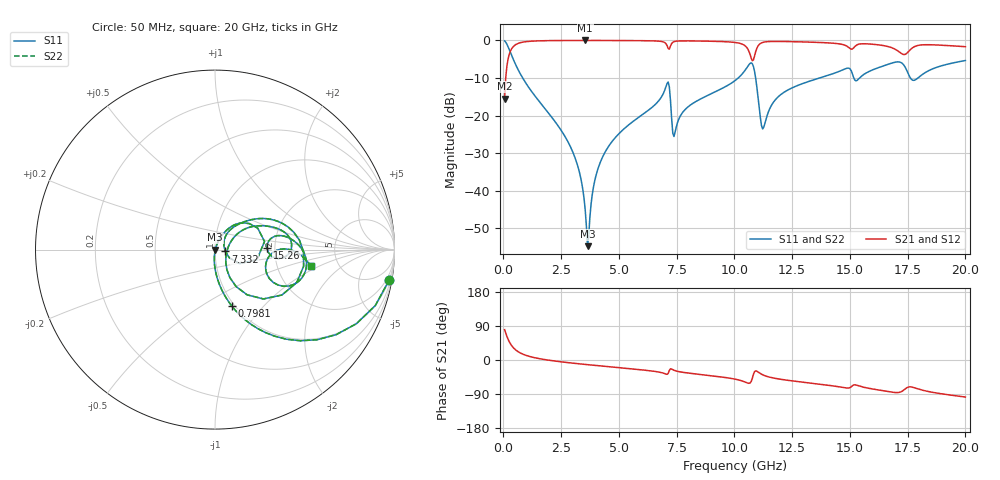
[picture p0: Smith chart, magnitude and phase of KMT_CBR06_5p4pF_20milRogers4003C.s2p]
! Data measured by Modelithics Inc. support@modelithics.com 813-866-6335
! KEMET CBR0603 5.4pF, Pad Width= 0.851mm, Pad Length= 0.64mm, Pad Gap= 0.62mm, 20mil Rogers 4003C substrate Data, January 2022
# hz S ma R 50
! 2 Port Network Data from SP1.SP block
! freq  magS11  angS11  magS21  angS21  magS12  angS12  magS22  angS22
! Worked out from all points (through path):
!   401 points, 50 MHz to 20 GHz, reference 50 ohm
!   highest |S21| = -0.02 dB at 3.541 GHz (marker M1); lowest = -15.5 dB at 50 MHz (marker M2)
!   group delay of S21, straight-line fit = 15.3 ps
!   lowest |S11| = -54.7 dB at 3.641 GHz (marker M3), VSWR 1.00, Z = 50.2 - j0.0924 ohm
!   |S11| at or under -10 dB: 833 MHz to 10.16 GHz (9.33 GHz wide, 170 % of centre); 10.92 GHz to 13.68 GHz (2.766 GHz wide, 22.5 % of centre); 17.62 GHz to 17.95 GHz (322.8 MHz wide, 1.82 % of centre)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
!   |S22| runs from -54.7 to -0.1 dB; largest |S21 - S12| = 0
!   S11 on the Smith chart (normalised r, x): 50 MHz: 1, -11; 798.1 MHz: 0.97, -0.69; 7.332 GHz: 1.12, -0.02; 15.26 GHz: 1.81, +0.04; 20 GHz: 3.13, -0.79
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5e7  0.9856 -9.9  0.1686 80.1  0.1686 80.1  0.9856 -9.9
2.99375e8  0.696 -46.9  0.7174 43.1  0.7174 43.1  0.696 -46.9
7.98125e8  0.3298 -73.3  0.9431 16.5  0.9431 16.5  0.3298 -73.3
2.74325e9  0.04784 -94.7  0.9972 -6.6  0.9972 -6.6  0.04784 -94.7
3.391625e9  0.01259 -93.1  0.9981 -10.8  0.9981 -10.8  0.01259 -93.1
3.54125e9  0.005519 -83.5  0.9981 -11.7  0.9981 -11.7  0.005519 -83.5
3.641e9  0.001836 -30.1  0.9981 -12.3  0.9981 -12.3  0.001836 -30.1
3.990125e9  0.01525 68.7  0.9979 -14.4  0.9979 -14.4  0.01525 68.7
4.439e9  0.03432 69.7  0.9973 -17.0  0.9973 -17.0  0.03432 69.7
6.73325e9  0.159 54.5  0.9769 -31.8  0.9769 -31.8  0.159 54.5
7.082375e9  0.2663 26.6  0.8553 -37.8  0.8553 -37.8  0.2663 26.6
7.33175e9  0.05828 -10.4  0.9434 -25.6  0.9434 -25.6  0.05828 -10.4
1.0025e10  0.292 36.1  0.9389 -50.5  0.9389 -50.5  0.292 36.1
1.052375e10  0.4266 17.1  0.8122 -59.7  0.8122 -59.7  0.4266 17.1
1.077312e10  0.4909 -22.0  0.5366 -48.8  0.5366 -48.8  0.4909 -22.0
1.127188e10  0.07013 3.3  0.9477 -40.4  0.9477 -40.4  0.07013 3.3
1.192025e10  0.1808 35.3  0.9688 -50.1  0.9688 -50.1  0.1808 35.3
1.336662e10  0.2946 26.9  0.9465 -61.5  0.9465 -61.5  0.2946 26.9
1.526188e10  0.2897 2.1  0.8542 -65.9  0.8542 -65.9  0.2897 2.1
1.670825e10  0.4874 -0.3  0.8192 -83.9  0.8192 -83.9  0.4874 -0.3
1.775562e10  0.2939 -14.3  0.8131 -72.6  0.8131 -72.6  0.2939 -14.3
2e10  0.5402 -9.5  0.8245 -97.7  0.8245 -97.7  0.5402 -9.5
